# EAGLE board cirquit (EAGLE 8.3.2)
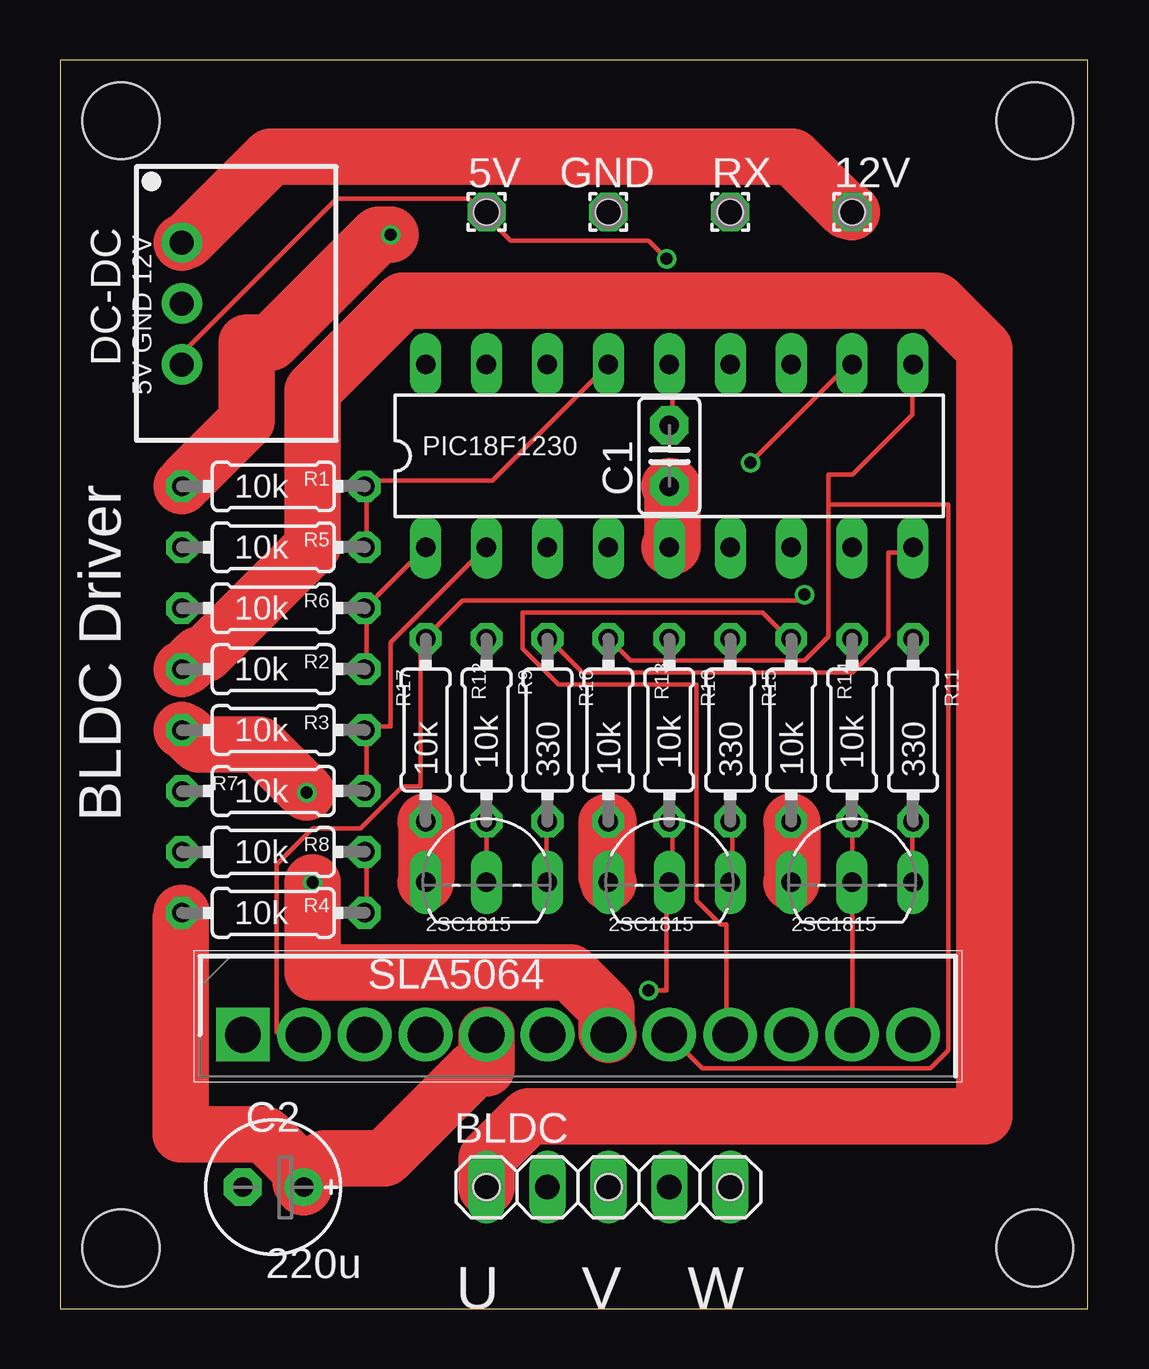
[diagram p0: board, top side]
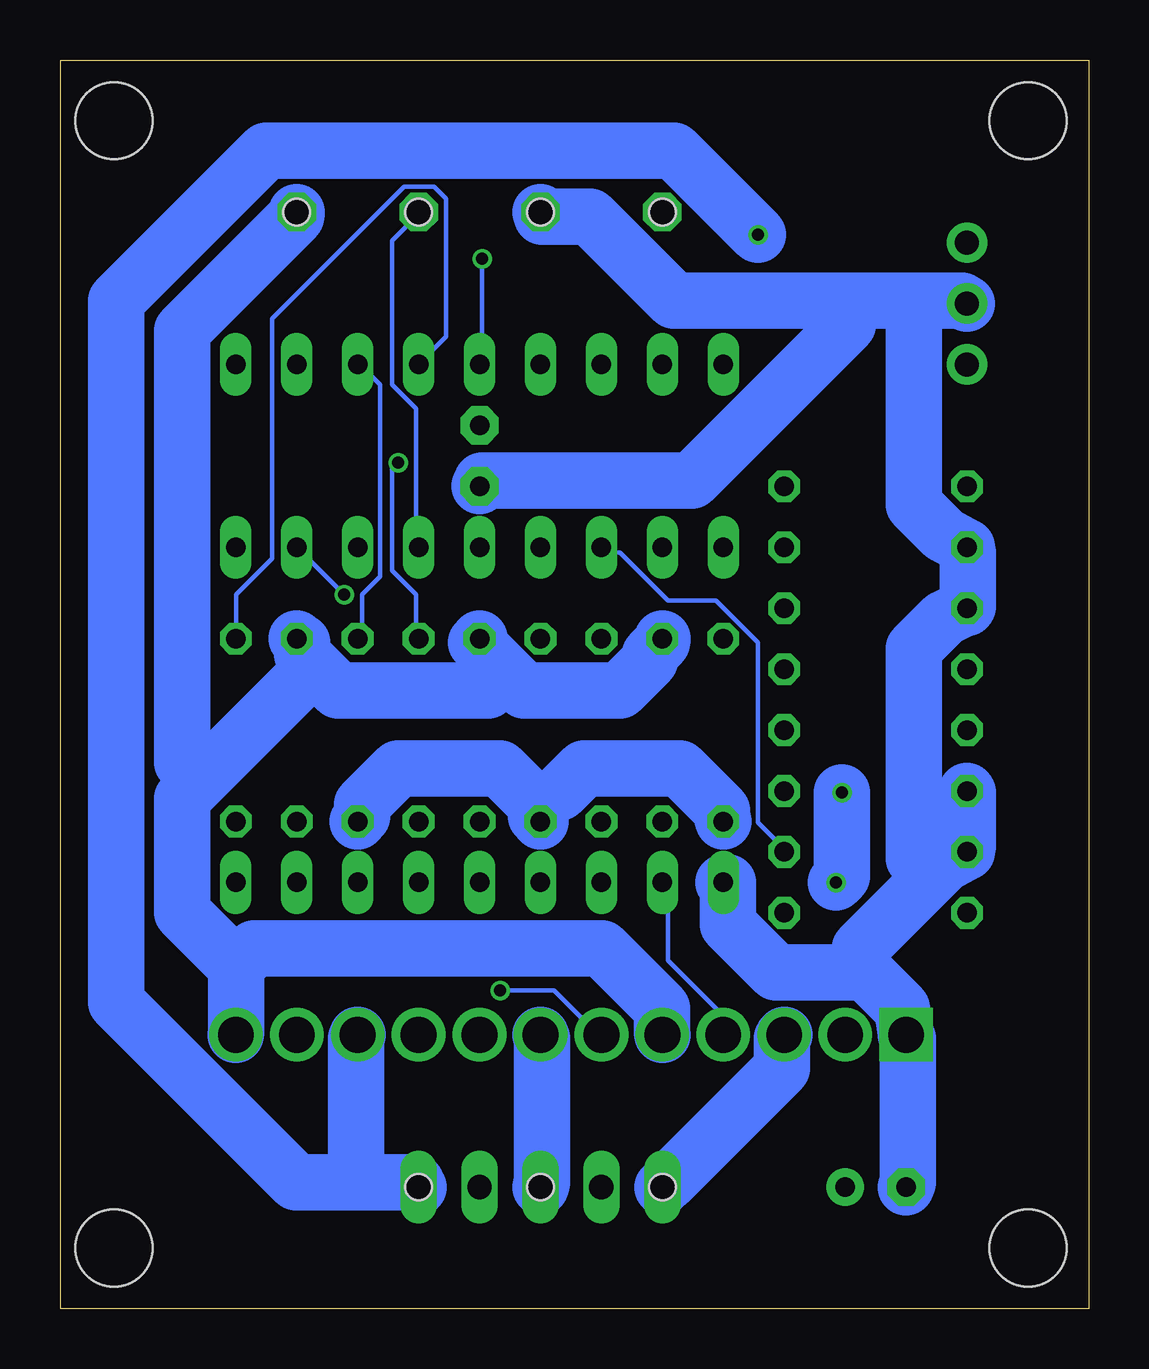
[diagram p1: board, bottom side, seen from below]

Size 42.85 x 52.06 mm. Coordinates in mm from the lower left corner, seen from the top.
Outline: 0,0 42.85,0 42.85,52.06 0,52.06 0,0
Copper layers (1*16): Top 0.035mm / dielectric 1.5mm / Bottom 0.035mm
Design rules "SeeedStudio_2layer_DRU_no_angle_20140221": minimum track width 6mil, minimum drill 12mil, track to track 6mil, track to pad 6mil, pad to pad 6mil, via to via 6mil, smd to smd 0mil, copper to edge 10mil, drill to drill 10mil, minimum pad ring 10mil, minimum via ring 6mil, stop-mask expansion 2mil, vias tented up to drill 100mil, thermal gap 10mil
Net classes: 0 default: width 0.178 mm, drill 0.5 mm, clearance 0.152 mm; 1 power: width 2.35 mm, drill 0.5 mm, clearance 0.152 mm; 2 GND: width 2.35 mm, drill 0.5 mm, clearance 0.152 mm
Holes 3.2 mm at 2.54,2.54 40.64,2.54 40.64,49.53 2.54,49.53
Holes 1.1 mm at 17.78,45.72 22.86,45.72 27.94,45.72 33.02,45.72 27.94,5.08 22.86,5.08 17.78,5.08

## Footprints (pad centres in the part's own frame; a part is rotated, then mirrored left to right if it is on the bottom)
1,6/0,8 = drill 0.813 pad 1.6 octagon: 1 0,0
1X05 = drill 1.016 long: 1 -5.08,0; 2 -2.54,0; 3 0,0; 4 2.54,0; 5 5.08,0
C2.5-2 = drill 0.813 pad 1.6 octagon: 1 -1.27,0; 2 1.27,0
E2,5-6E = drill 0.813 pad 1.575: + -1.27,0 | drill 0.813 pad 1.575 octagon: - 1.27,0
SIP3 = drill 1 pad 1.676: 1 -2.54,0; 2 0,0; 3 2.54,0
DIL18 = drill 0.813 long: 1 -10.16,-3.81; 2 -7.62,-3.81; 3 -5.08,-3.81; 4 -2.54,-3.81; 5 0,-3.81; 6 2.54,-3.81; 7 5.08,-3.81; 8 7.62,-3.81; 9 10.16,-3.81; 10 10.16,3.81; 11 7.62,3.81; 12 5.08,3.81; 13 2.54,3.81; 14 0,3.81; 15 -2.54,3.81; 16 -5.08,3.81; 17 -7.62,3.81; 18 -10.16,3.81
0204/7 = drill 0.813 octagon: 1 -3.81,0; 2 3.81,0
TO254P500X3150X1890-12P = drill 1.49 pad 2.235 square: 1 0,0 | drill 1.49 pad 2.235: 2 2.54,0; 3 5.08,0; 4 7.62,0; 5 10.16,0; 6 12.7,0; 7 15.24,0; 8 17.78,0; 9 20.32,0; 10 22.86,0; 11 25.4,0; 12 27.94,0
TO92-ECB = drill 0.813 long: B 2.54,0; C 0,0; E -2.54,0

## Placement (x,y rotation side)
5V  [1,6/0,8]  17.78,45.72 0 top
12V  [1,6/0,8]  33.02,45.72 0 top
BLDC  [1X05]  22.86,5.08 0 top
C1  0.1u  [C2.5-2]  25.4,35.56 90 top
C2  220u  [E2,5-6E]  8.89,5.08 180 top
DC-DC  R-78C1.8-1.0  [SIP3]  5.08,41.91 270 top
GND  [1,6/0,8]  22.86,45.72 0 top
PIC18F1230  PIC18F1220P  [DIL18]  25.4,35.56 0 top
R1  10k  [0204/7]  8.89,34.29 0 top
R2  10k  [0204/7]  8.89,26.67 0 top
R3  10k  [0204/7]  8.89,24.13 0 top
R4  10k  [0204/7]  8.89,16.51 0 top
R5  10k  [0204/7]  8.89,31.75 0 top
R6  10k  [0204/7]  8.89,29.21 0 top
R7  10k  [0204/7]  8.89,21.59 0 top
R8  10k  [0204/7]  8.89,19.05 0 top
R9  330  [0204/7]  20.32,24.13 270 top
R10  330  [0204/7]  27.94,24.13 270 top
R11  330  [0204/7]  35.56,24.13 270 top
R12  10k  [0204/7]  17.78,24.13 90 top
R13  10k  [0204/7]  25.4,24.13 90 top
R14  10k  [0204/7]  33.02,24.13 90 top
R15  10k  [0204/7]  30.48,24.13 270 top
R16  10k  [0204/7]  22.86,24.13 270 top
R17  10k  [0204/7]  15.24,24.13 270 top
RX  [1,6/0,8]  27.94,45.72 0 top
SLA5064  SLA5064  [TO254P500X3150X1890-12P]  7.62,11.43 0 top
T1  2SC1815  [TO92-ECB]  17.78,17.78 0 top
T2  2SC1815  [TO92-ECB]  25.4,17.78 0 top
T3  2SC1815  [TO92-ECB]  33.02,17.78 0 top

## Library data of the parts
5V 12V GND RX = wirepad
BLDC = pinhead
C1 = capacitor-wima
C2 R1-R17 = resistor
DC-DC = dc-dc-converter
PIC18F1230 = microchip; MF: MICROCHIP; MPN: PIC18F1220-I/P; OC_FARNELL: 9761977; OC_NEWARK: 92C2429
SLA5064 = SLA5064; DESCRIPTION: N-channel+P-channel 3-phase motor drive; HEIGHT: 5mm; MANUFACTURER_NAME: Sanken; MANUFACTURER_PART_NUMBER: SLA5064; SUPPLIER_NAME: RS
T1-T3 = transistor

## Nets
+12V [power]: 12V.1 C2.+ DC-DC.1 R4.1 R12.2 R13.2 R14.2 SLA5064.5 SLA5064.12
GND [GND]: C1.1 C2.- DC-DC.2 GND.1 PIC18F1230.5 R5.1 R6.1 R7.1 R8.1 R15.2 R16.2 R17.2 SLA5064.1 T1.E T2.E T3.E
N$1: PIC18F1230.15 R1.2 R5.2
N$2: PIC18F1230.1 R2.2 R6.2
N$3: PIC18F1230.2 R3.2 R7.2
N$4: PIC18F1230.3 R4.2 R8.2
N$5: PIC18F1230.16
N$6 [power]: BLDC.1 R2.1 SLA5064.3
N$7 [power]: BLDC.3 R3.1 SLA5064.7
N$9: PIC18F1230.9 R9.1
N$10: PIC18F1230.11 R10.1
N$11: PIC18F1230.13 R11.1
N$12: R9.2 T1.B
N$13: R10.2 T2.B
N$14: R11.2 T3.B
N$15: R12.1 SLA5064.4 T1.C
N$16: R13.1 SLA5064.6 T2.C
N$17: R14.1 SLA5064.11 T3.C
N$18: PIC18F1230.7
N$19: PIC18F1230.4
N$20: PIC18F1230.17
N$21: PIC18F1230.18
N$22: PIC18F1230.8 R17.1 SLA5064.2
N$23: PIC18F1230.10 R16.1 SLA5064.8
N$24: PIC18F1230.12 R15.1 SLA5064.9
N$25: PIC18F1230.6 RX.1
N$26: 5V.1 C1.2 DC-DC.3 PIC18F1230.14
N$29 [power]: BLDC.5 R1.1 SLA5064.10

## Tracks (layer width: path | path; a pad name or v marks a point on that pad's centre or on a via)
+12V
  Top 2.35: 12V.1 32.79,45.77 30.54,48.02 8.79,48.02 5.29,44.52 DC-DC.1 | 10.04,5.77 8.54,7.27 5.04,7.27 5.04,16.27 R4.1 | 10.04,5.77 10.04,5.27 C2.+ | SLA5064.5 17.79,11.27 17.79,10.02 17.29,10.02 13.54,6.27 11.04,6.27 10.04,5.77
  Bottom 2.35: 24.29,26.52 25.54,27.77 R13.2 | 24.29,26.52 23.54,25.77 19.54,25.77 18.29,27.02 18.29,27.27 17.79,27.77 R12.2 | 32.29,26.77 31.29,25.77 25.04,25.77 24.29,26.52 | 32.29,26.77 32.79,27.27 32.79,27.77 R14.2 | 35.54,14.27 35.54,11.52 SLA5064.12 | 35.54,14.27 37.79,16.52 37.79,21.27 37.04,22.02 | 32.29,26.77 37.04,22.02 | SLA5064.5 17.79,11.52 17.79,12.52 20.29,15.02 34.79,15.02 35.54,14.27 | 12V.1 33.04,45.52 37.79,40.77 37.79,22.77 37.04,22.02
GND
  Top 2.35: PIC18F1230.5 25.54,31.77 25.54,34.27 C1.1 | T2.E 22.79,18.02 22.79,20.27 R16.2 | T3.E 30.54,18.02 30.54,20.27 R15.2 | T1.E 15.29,18.02 15.29,20.27 R17.2
  Bottom 2.35: 5.04,29.27 5.04,31.52 R5.1 6.04,32.27 7.29,33.52 7.29,42.02 | 5.04,29.27 R6.1 | 7.29,42.02 5.29,42.02 DC-DC.2 | 7.29,42.02 10.04,42.02 | 10.04,42.02 17.29,42.02 20.79,45.52 22.79,45.52 GND.1 | C1.1 25.29,34.52 16.54,34.52 10.04,41.02 10.04,42.02 | 23.04,21.02 23.04,20.52 R16.2 | 23.04,21.02 24.54,22.52 28.79,22.52 30.29,21.02 30.29,20.52 R15.2 | R7.1 5.04,21.52 5.04,19.27 R8.1 6.04,18.52 6.54,18.02 | C2.- 7.54,5.27 7.54,11.27 SLA5064.1 7.79,12.52 9.29,14.02 9.54,14.02 | 9.54,14.02 13.04,14.02 15.04,16.02 15.04,17.77 T1.E | 6.54,18.02 9.54,15.02 9.54,14.02 | 23.04,21.02 22.04,21.52 21.04,22.52 17.04,22.52 15.29,20.77 15.29,20.52 R17.2 | 5.04,29.27 6.04,28.77 7.29,27.52 7.29,18.77 6.54,18.02
N$1
  Top 0.178: R5.2 12.79,31.77 12.79,34.27 R1.2 12.79,34.52 18.04,34.52 22.79,39.27 PIC18F1230.15
N$2
  Top 0.178: R2.2 12.79,26.77 12.79,29.02 R6.2 12.79,29.27 15.04,31.52 PIC18F1230.1
N$3
  Top 0.178: R7.2 12.79,21.77 12.79,24.02 R3.2 12.79,24.27 13.79,24.27 13.79,27.77 17.54,31.52 PIC18F1230.2
N$4
  Top 0.178: R4.2 12.79,16.52 12.79,19.02 R8.2
  Bottom 0.178: PIC18F1230.3 20.29,31.52 19.54,31.52 17.54,29.52 15.54,29.52 13.79,27.77 13.79,20.27 12.79,19.27 R8.2
N$6
  Top 2.35: R2.1 5.29,26.77 5.79,27.27 6.04,27.27 10.54,31.77 10.54,38.27 14.29,42.02 36.54,42.02 38.54,40.02 38.54,8.02 19.54,8.02 17.79,6.27 17.79,5.27 BLDC.1
  Bottom 2.35: SLA5064.3 12.79,11.27 12.79,10.02 17.54,5.27 BLDC.1
N$7  (via drill 0.5)
  Top 2.35: v10.29,21.52 8.29,23.52 5.79,23.52 5.29,24.02 R3.1 | v10.54,17.77 10.54,14.02 21.29,14.02 22.79,12.52 22.79,11.52 SLA5064.7
  Bottom 2.35: v10.29,21.52 10.29,18.02 v10.54,17.77 | BLDC.3 22.79,5.27 22.79,11.27 SLA5064.7
N$9
  Top 0.178: R9.1 20.54,27.77 21.79,26.52 33.04,26.52 34.54,28.02 34.54,31.52 35.54,31.52 PIC18F1230.9
N$10  (via drill 0.5)
  Top 0.178: v28.79,35.27 32.79,39.27 PIC18F1230.11
  Bottom 0.178: v28.79,35.27 29.04,35.02 29.04,30.77 28.04,29.77 28.04,28.02 R10.1
N$11
  Bottom 0.178: PIC18F1230.13 26.79,40.52 26.79,46.27 27.29,46.77 28.54,46.77 34.04,41.27 34.04,31.27 35.54,29.77 35.54,28.02 R11.1
N$12
  Top 0.178: T1.B 20.29,18.02 20.29,20.27 R9.2
N$13
  Top 0.178: T2.B 28.04,18.02 28.04,20.27 R10.2
N$14
  Top 0.178: T3.B 35.54,18.02 35.54,20.27 R11.2
N$15
  Top 0.178: T1.C 17.79,18.02 17.79,20.27 R12.1
  Bottom 0.178: T1.C 17.54,17.77 17.54,14.52 15.29,12.27 15.29,11.52 SLA5064.4
N$16  (via drill 0.5)
  Top 0.178: R13.1 25.54,20.27 25.54,18.02 T2.C 25.29,17.77 25.29,13.27 v24.54,13.27
  Bottom 0.178: v24.54,13.27 22.29,13.27 20.54,11.52 SLA5064.6
N$17
  Top 0.178: R14.1 33.04,20.27 33.04,18.02 T3.C 33.04,17.77 33.04,11.52 SLA5064.11
N$22  (via drill 0.5)
  Top 0.178: SLA5064.2 10.04,11.52 9.04,11.52 9.04,18.52 10.54,20.02 12.54,20.02 14.29,21.77 15.04,21.77 15.04,27.77 R17.1 15.29,28.02 16.79,29.52 30.79,29.52 v31.04,29.77
  Bottom 0.178: v31.04,29.77 PIC18F1230.8
N$23
  Top 0.178: 32.04,33.52 32.04,34.77 33.04,34.77 35.54,37.27 35.54,39.27 PIC18F1230.10 | 32.04,33.52 32.04,28.02 31.04,27.02 23.79,27.02 23.04,27.77 R16.1 | 32.04,33.52 37.04,33.52 37.04,10.77 36.29,10.02 26.79,10.02 25.54,11.27 SLA5064.8
N$24
  Top 0.178: SLA5064.9 27.79,11.52 27.79,16.02 27.54,16.02 26.54,17.02 26.54,26.02 20.79,26.02 19.29,27.52 19.29,29.02 29.29,29.02 30.29,28.02 R15.1
  Bottom 0.178: R15.1 30.29,28.02 30.29,29.77 29.54,30.52 29.54,38.52 30.29,39.27 PIC18F1230.12
N$25
  Bottom 0.178: PIC18F1230.6 28.04,31.77 28.04,37.52 29.04,38.52 29.04,44.52 28.04,45.52 RX.1
N$26  (via drill 0.5)
  Top 0.178: PIC18F1230.14 25.54,39.27 25.54,37.02 C1.2 | DC-DC.3 5.29,39.52 5.29,40.02 11.54,46.27 17.04,46.27 17.54,45.77 5V.1 17.79,45.52 18.79,44.52 24.54,44.52 v25.29,43.77
  Bottom 0.178: v25.29,43.77 25.29,39.52 PIC18F1230.14
N$29  (via drill 0.5)
  Top 2.35: v13.79,44.77 13.29,44.77 8.79,40.27 7.79,40.27 7.79,37.02 5.29,34.52 R1.1
  Bottom 2.35: v13.79,44.77 17.29,48.27 34.29,48.27 40.54,42.02 40.54,12.77 33.04,5.27 30.54,5.27 | 30.54,5.27 28.04,5.27 BLDC.5 | 30.54,5.27 30.54,11.27 SLA5064.10

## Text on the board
tNames: 5V GND 12V | BLDC Driver | U V W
